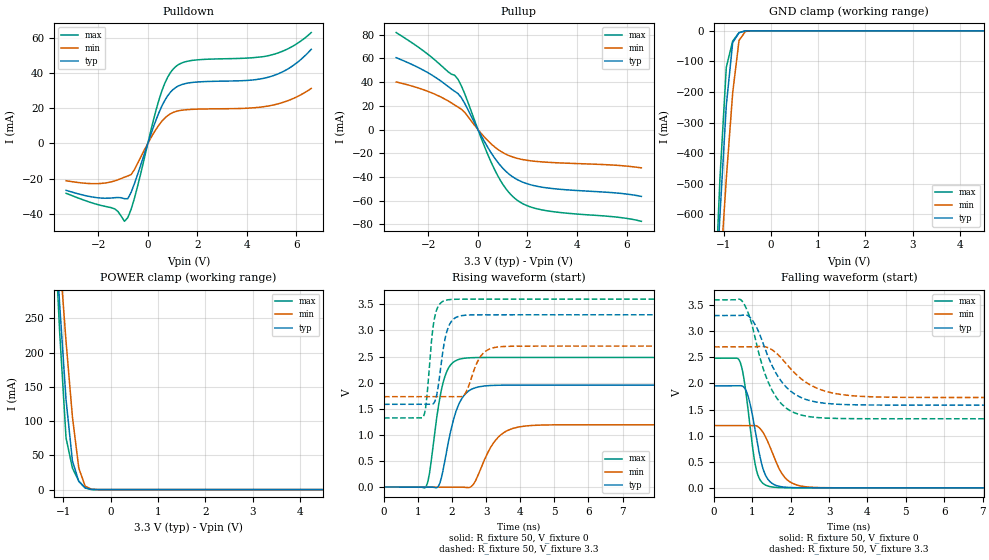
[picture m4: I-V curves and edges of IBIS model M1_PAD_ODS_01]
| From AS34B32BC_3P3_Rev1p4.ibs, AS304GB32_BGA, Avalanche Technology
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[Model] M1_PAD_ODS_01
Model_type I/O
Enable   Active-High
Vinl  =  0.8
Vinh  =  2.2
Vmeas =  1.65
Cref  =  30e-12
| Capacitance  typ   min   max
C_comp   6.058162e-12   5.681079e-12   6.591827e-12
| Variables   typ   min   max
[GND Clamp Reference]   0   0   0
[POWER Clamp Reference]   3.3   2.7   3.6
[Pulldown Reference]   0   0   0
[Pullup Reference]   3.3   2.7   3.6
[Temperature Range]   25   125   -40
[Voltage Range]   3.3   2.7   3.6
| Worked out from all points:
|   slope of the pulldown table from 0 to 0.495 V, typ, clamps not added: 26.1 ohm
|   slope of the pullup table from 0 to 0.495 V, typ, clamps not added: 27 ohm
|   GND clamp passes 1 mA (typ) near -0.55 V on its own axis
|   POWER clamp passes 1 mA (typ) near -0.44 V on its own axis
|   falling waveform, R_fixture 50, V_fixture 0: 20-80 % time 313ps typ, 446ps min, 260ps max; typ from 1.95 V to 0 V
|   falling waveform, R_fixture 50, V_fixture 3.3: 20-80 % time 705ps typ, 902ps min, 602ps max; typ from 3.3 V to 1.58 V
|   rising waveform, R_fixture 50, V_fixture 0: 20-80 % time 426ps typ, 583ps min, 344ps max; typ from 0 V to 1.95 V
|   rising waveform, R_fixture 50, V_fixture 3.3: 20-80 % time 244ps typ, 361ps min, 192ps max; typ from 1.58 V to 3.3 V
[GND Clamp]
| Voltage   I(typ)   I(min)   I(max)
-3.3V     -7.845A    -6.789A    -9.429A
-1.21V    -1.003A    -1.135A    -970mA
-1.076V   -602.2mA   -800.5mA   -482.6mA
-941.4mV  -243.3mA   -483.1mA   -119mA
-806.9mV  -38.59mA   -202.8mA   -33.75mA
-672.4mV  -6.344mA   -31.46mA   -5.83mA
-537.9mV  -287.2uA   -2.017mA   -75.02uA
-403.4mV  -2.377uA   -74.3uA    -149.1nA
6.6V      0A         0A         0A
[POWER Clamp]
| Voltage   I(typ)   I(min)   I(max)
-3.3V     3.089A     2.693A     3.722A
-1.21V    423.7mA    470.3mA    418.3mA
-1.076V   269.4mA    340.2mA    228.7mA
-941.4mV  130.8mA    215.7mA    75.29mA
-806.9mV  41.91mA    106.1mA    31.39mA
-672.4mV  11.9mA     31.42mA    12.43mA
-537.9mV  2.843mA    4.992mA    2.292mA
-403.4mV  242.8uA    643.4uA    36.75uA
-269mV    569.5nA    24.47uA    93.03nA
6.6V      0A         0A         0A
[Pulldown]
| Voltage   I(typ)   I(min)   I(max)
-3.3V     -26.68mA   -21.22mA   -28.37mA
-1.345V   -30.89mA   -21.35mA   -37.2mA
-941.4mV  -31.46mA   -19.19mA   -44.32mA
-806.9mV  -31.44mA   -18.5mA    -42.21mA
-537.9mV  -22.81mA   -14.83mA   -31.1mA
455.2mV   17.74mA    10.61mA    25.04mA
682.8mV   24.44mA    14.41mA    34.16mA
1.024V    30.75mA    17.67mA    42.38mA
1.821V    34.78mA    19.45mA    47.35mA
4.914V    37.93mA    21.47mA    50.14mA
5.783V    43.54mA    25.06mA    54.82mA
6.6V      53.61mA    31.34mA    63.15mA
[Pullup]
| Voltage   I(typ)   I(min)   I(max)
-3.3V     60.61mA    40.12mA    81.78mA
-1.883V   46.22mA    31.07mA    61.18mA
-806.9mV  30.34mA    18.97mA    42.44mA
-537.9mV  22.21mA    14.55mA    30.44mA
227.6mV   -8.868mA   -5.574mA   -12.38mA
682.8mV   -24.26mA   -14.79mA   -34.2mA
1.138V    -35.44mA   -20.91mA   -50.18mA
1.593V    -42.28mA   -24.34mA   -59.75mA
2.048V    -46.13mA   -26.16mA   -64.77mA
2.731V    -49.08mA   -27.51mA   -68.35mA
5.659V    -53.66mA   -30.27mA   -74.01mA
6.6V      -56.41mA   -32.34mA   -77.42mA
[Ramp]
dV/dt_r   1.17185/0.42631n  0.715782/0.582767n  1.4895/0.344067n
dV/dt_f   1.02933/0.70453n  0.581576/0.901957n  1.3662/0.60195n
R_load = 50
[Falling Waveform]
R_fixture = 50
V_fixture = 0
V_fixture_min = 0
V_fixture_max = 0
| Time   V(typ)   V(min)   V(max)
0s        1.953V     1.193V     2.482V
665.2ps   1.956V     1.194V     2.433V
754.1ps   1.944V     1.194V     2.193V
870.3ps   1.795V     1.194V     1.598V
1.104ns   964.2mV    1.188V     339.8mV
1.293ns   328.9mV    1.042V     74.68mV
1.531ns   77.68mV    651.1mV    14.73mV
1.909ns   9.553mV    152.1mV    1.649mV
2.629ns   926uV      8.132mV    831.5uV
21.88ns   -336.7nV   439.8nV    13.87nV
[Falling Waveform]
R_fixture = 50
V_fixture = 3.3
V_fixture_min = 2.7
V_fixture_max = 3.6
| Time   V(typ)   V(min)   V(max)
0s        3.3V       2.7V       3.6V
737.6ps   3.308V     2.701V     3.572V
1.049ns   3.154V     2.702V     2.939V
1.276ns   2.771V     2.709V     2.298V
1.511ns   2.342V     2.646V     1.869V
1.897ns   1.918V     2.364V     1.519V
2.455ns   1.679V     1.994V     1.366V
3.313ns   1.598V     1.788V     1.328V
4.577ns   1.585V     1.736V     1.324V
21.88ns   1.584V     1.731V     1.323V
[Rising Waveform]
R_fixture = 50
V_fixture = 0
V_fixture_min = 0
V_fixture_max = 0
| Time   V(typ)   V(min)   V(max)
0s        28.83nV    251.3nV    41.19nV
1.229ns   -652.1uV   -346.3uV   3.046mV
1.592ns   11.16mV    -448.6uV   1.521V
1.769ns   441.9mV    -498.8uV   2.08V
2.048ns   1.309V     -577.2uV   2.397V
2.336ns   1.743V     -4.578mV   2.466V
2.622ns   1.889V     49.83mV    2.479V
3.364ns   1.95V      962.3mV    2.482V
4.141ns   1.953V     1.168V     2.482V
21.88ns   1.953V     1.193V     2.482V
[Rising Waveform]
R_fixture = 50
V_fixture = 3.3
V_fixture_min = 2.7
V_fixture_max = 3.6
| Time   V(typ)   V(min)   V(max)
0s        1.584V     1.731V     1.323V
1.158ns   1.585V     1.731V     1.351V
1.241ns   1.585V     1.731V     1.613V
1.407ns   1.584V     1.731V     2.873V
1.493ns   1.64V      1.731V     3.267V
1.86ns    3.009V     1.732V     3.586V
2.335ns   3.289V     1.753V     3.599V
2.853ns   3.299V     2.519V     3.6V
3.499ns   3.3V       2.692V     3.6V
21.88ns   3.3V       2.7V       3.6V
